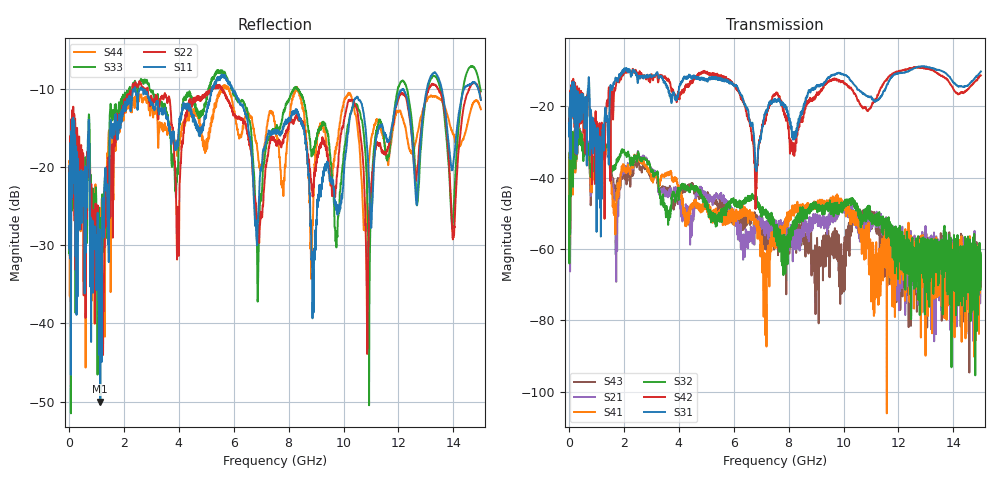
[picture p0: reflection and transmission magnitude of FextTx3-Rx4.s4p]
!  = SDD11
!  = SDD12
!  = SDC11
!  = SDC12
!  = SDD21
!  = SDD22
!  = SDC12
!  = SDC22
!  = SCD11
!  = SCD12
!  = SCC11
!  = SCC12
!  = SCD21
!  = SCD22
!  = SCC21
!  = SCC22
! FILE: N:\QM 2007\Prüfprotokolle\Highspeed\Konfektionierte Ltg\L45593-D106\D30\8216\0002\Fext\FextTx3-Rx4.s4p
# MHz S RI R 50.00
! FREQ  S11  S12  S13  S14
!  S21  S22  S23  S24
!  S31  S32  S33  S34
!  S41  S42  S43  S44
!  REAL  IMAG  REAL  IMAG  REAL  IMAG  REAL  IMAG
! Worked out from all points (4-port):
!   2999 points, 10 MHz to 15 GHz, reference 50 ohm
!   strongest paths, dB at 10 MHz, 3.755 GHz, 7.505 GHz, 11.26 GHz, 15 GHz:
!     S31: -24.8, -17.1, -18.3, -18.3, -10.3
!     S42: -23.8, -15.3, -17.0, -16.9, -11.4
!     S32: -45.2, -45.8, -55.0, -52.2, -65.2
!     S41: -44.8, -40.8, -57.3, -61.2, -62.3
!     S21: -40.6, -46.1, -54.2, -52.9, -65.0
!     S43: -43.1, -46.1, -55.8, -54.0, -65.6
!   lowest |S11| = -50.0 dB at 1.145 GHz (marker M1), VSWR 1.01, Z = 49.7 + j0.0529 ohm
!   |S11| at or under -10 dB: start of sweep to 2.363 GHz; 2.698 GHz to 5.195 GHz (2.497 GHz wide, 63.3 % of centre); 5.964 GHz to 12.14 GHz (6.18 GHz wide, 68.3 % of centre)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
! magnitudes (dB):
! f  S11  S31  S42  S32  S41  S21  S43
! 10 MHz  -19.9  -24.8  -23.8  -45.2  -44.8  -40.6  -43.1
! 1.145 GHz  -50.0  -48.5  -27.6  -34.6  -34.7  -34.0  -34.5
! 2.05 GHz  -12.2  -9.8  -10.5  -33.3  -38.1  -38.2  -39.7
! 5.885 GHz  -9.4  -13.6  -13.2  -47.2  -50.1  -48.8  -50.5
! 6.81 GHz  -27.4  -37.4  -45.1  -46.7  -52.0  -53.7  -52.0
! 7.53 GHz  -15.2  -18.6  -16.7  -56.6  -56.9  -54.4  -56.3
! 15 GHz  -11.4  -10.3  -11.4  -65.2  -62.3  -65.0  -65.6
